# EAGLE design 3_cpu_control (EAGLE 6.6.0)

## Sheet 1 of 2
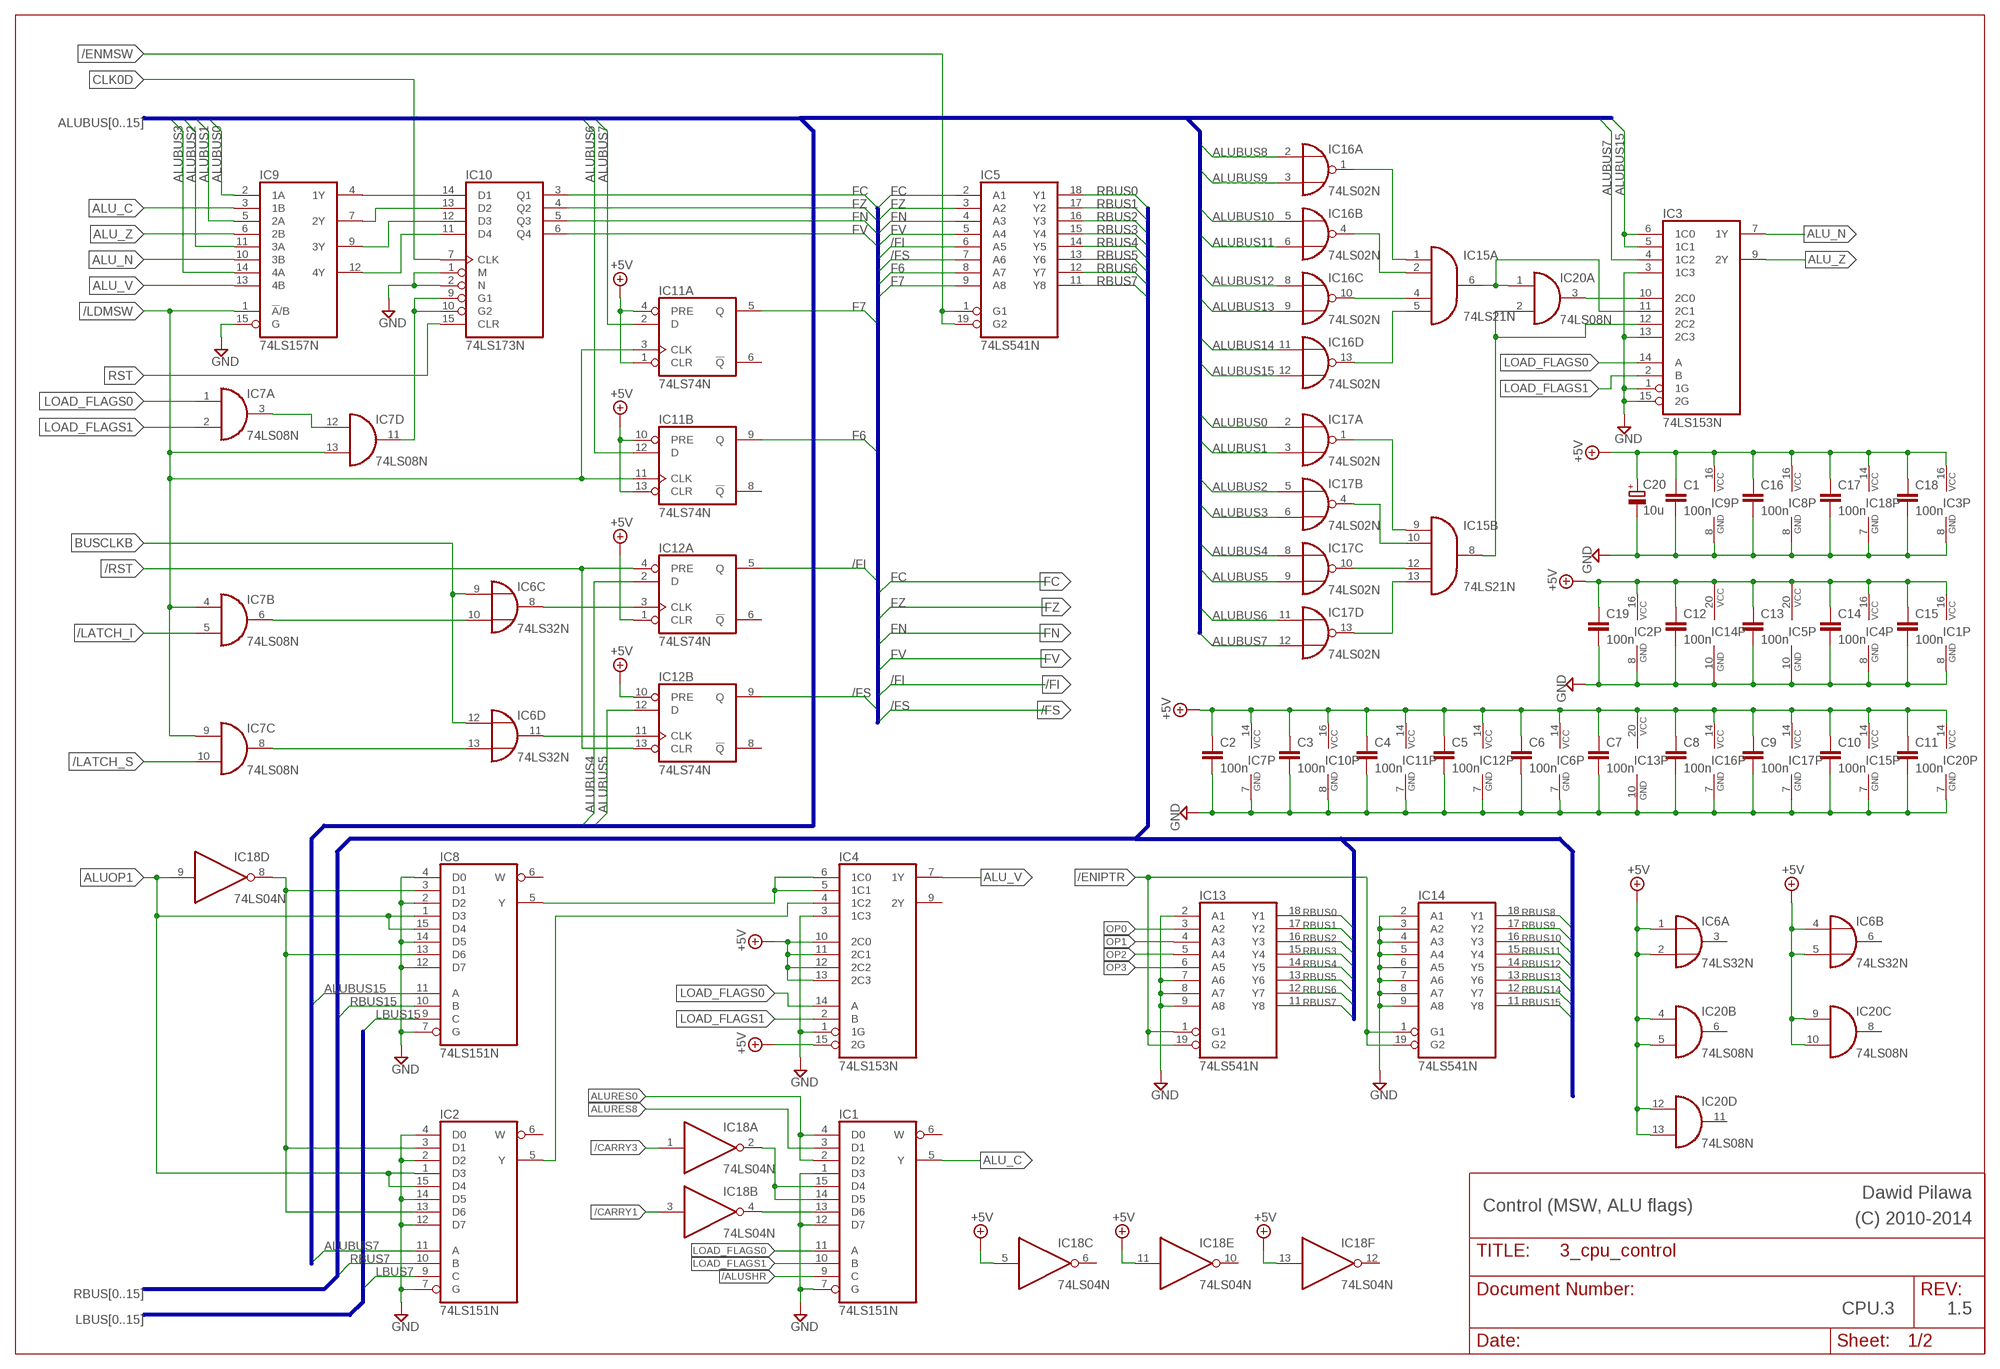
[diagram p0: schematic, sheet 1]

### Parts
C1  100n  C-EU050-024X044  [C050-024X044]
C2  100n  C-EU050-024X044  [C050-024X044]
C3  100n  C-EU050-024X044  [C050-024X044]
C4  100n  C-EU050-024X044  [C050-024X044]
C5  100n  C-EU050-024X044  [C050-024X044]
C6  100n  C-EU050-024X044  [C050-024X044]
C7  100n  C-EU050-024X044  [C050-024X044]
C8  100n  C-EU050-024X044  [C050-024X044]
C9  100n  C-EU050-024X044  [C050-024X044]
C10  100n  C-EU050-024X044  [C050-024X044]
C11  100n  C-EU050-024X044  [C050-024X044]
C12  100n  C-EU050-024X044  [C050-024X044]
C13  100n  C-EU050-024X044  [C050-024X044]
C14  100n  C-EU050-024X044  [C050-024X044]
C15  100n  C-EU050-024X044  [C050-024X044]
C16  100n  C-EU050-024X044  [C050-024X044]
C17  100n  C-EU050-024X044  [C050-024X044]
C18  100n  C-EU050-024X044  [C050-024X044]
C19  100n  C-EU050-024X044  [C050-024X044]
C20  10u  CPOL-EUE2.5-6  [E2,5-6]
IC1  74LS151N  [DIL16]
IC2  74LS151N  [DIL16]
IC3  74LS153N  [DIL16]
IC4  74LS153N  [DIL16]
IC5  74LS541N  [DIL20]
IC6  74LS32N  [DIL14]
IC7  74LS08N  [DIL14]
IC8  74LS151N  [DIL16]
IC9  74LS157N  [DIL16]
IC10  74LS173N  [DIL16]
IC11  74LS74N  [DIL14]
IC12  74LS74N  [DIL14]
IC13  74LS541N  [DIL20]
IC14  74LS541N  [DIL20]
IC15  74LS21N  [DIL14]
IC16  74LS02N  [DIL14]
IC17  74LS02N  [DIL14]
IC18  74LS04N  [DIL14]
IC20  74LS08N  [DIL14]

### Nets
+5V: C1.1 C2.1 C3.1 C4.1 C5.1 C6.1 C7.1 C8.1 C9.1 C10.1 C11.1 C12.1 C13.1 C14.1 C15.1 C16.1 C17.1 C18.1 C19.1 C20.+ IC1.16(VCC) IC2.16(VCC) IC3.16(VCC) IC4.10(2C0) IC4.11(2C1) IC4.12(2C2) IC4.13(2C3) IC4.15(2G) IC4.16(VCC) IC5.20(VCC) IC6.1(A:I0) IC6.2(A:I1) IC6.4(B:I0) IC6.5(B:I1) IC6.14(P:VCC) IC7.14(P:VCC) IC8.16(VCC) IC9.16(VCC) IC10.16(VCC) IC11.1(A:CLR) IC11.4(A:PRE) IC11.10(B:PRE) IC11.13(B:CLR) IC11.14(P:VCC) IC12.1(A:CLR) IC12.10(B:PRE) IC12.14(P:VCC) IC13.20(VCC) IC14.20(VCC) IC15.14(P:VCC) IC16.14(P:VCC) IC17.14(P:VCC) IC18.5(C:I) IC18.11(E:I) IC18.13(F:I) IC18.14(P:VCC) IC20.4(B:I0) IC20.5(B:I1) IC20.9(C:I0) IC20.10(C:I1) IC20.12(D:I0) IC20.13(D:I1) IC20.14(P:VCC) ; also sheet 2
/ALUSHR: IC1.9(C) ; also sheet 2
/CARRY1: IC18.3(B:I) ; also sheet 2
/CARRY3: IC18.1(A:I) ; also sheet 2
/ENIPTR: IC13.1(G1) IC13.19(G2) IC14.1(G1) IC14.19(G2) ; also sheet 2
/ENMSW: IC5.1(G1) IC5.19(G2) ; also sheet 2
/FI: IC5.6(A5) IC12.5(A:Q) ; also sheet 2
/FS: IC5.7(A6) IC12.9(B:Q) ; also sheet 2
/LATCH_I: IC7.5(B:I1) ; also sheet 2
/LATCH_S: IC7.10(C:I1) ; also sheet 2
/LDMSW: IC7.4(B:I0) IC7.9(C:I0) IC7.13(D:I1) IC9.1(!A!/B) IC11.3(A:CLK) IC11.11(B:CLK) ; also sheet 2
/RST: IC12.4(A:PRE) IC12.13(B:CLR) ; also sheet 2
ALU_C: IC1.5(Y) IC9.3(1B)
ALU_N: IC3.7(1Y) IC9.10(3B)
ALU_V: IC4.7(1Y) IC9.13(4B)
ALU_Z: IC3.9(2Y) IC9.6(2B)
ALUBUS0: IC9.2(1A) IC17.2(A:I0) ; also sheet 2
ALUBUS1: IC9.5(2A) IC17.3(A:I1) ; also sheet 2
ALUBUS2: IC9.11(3A) IC17.5(B:I0) ; also sheet 2
ALUBUS3: IC9.14(4A) IC17.6(B:I1) ; also sheet 2
ALUBUS4: IC12.2(A:D) IC17.8(C:I0) ; also sheet 2
ALUBUS5: IC12.12(B:D) IC17.9(C:I1) ; also sheet 2
ALUBUS6: IC11.12(B:D) IC17.11(D:I0) ; also sheet 2
ALUBUS7: IC2.11(A) IC3.4(1C2) IC11.2(A:D) IC17.12(D:I1) ; also sheet 2
ALUBUS8: IC16.2(A:I0) ; also sheet 2
ALUBUS9: IC16.3(A:I1) ; also sheet 2
ALUBUS10: IC16.5(B:I0) ; also sheet 2
ALUBUS11: IC16.6(B:I1) ; also sheet 2
ALUBUS12: IC16.8(C:I0) ; also sheet 2
ALUBUS13: IC16.9(C:I1) ; also sheet 2
ALUBUS14: IC16.11(D:I0) ; also sheet 2
ALUBUS15: IC3.5(1C1) IC3.6(1C0) IC8.11(A) IC16.12(D:I1) ; also sheet 2
ALUOP1: IC2.1(D3) IC2.15(D4) IC8.1(D3) IC8.15(D4) IC18.9(D:I) ; also sheet 2
ALURES0: IC1.2(D2) IC1.4(D0) ; also sheet 2
ALURES8: IC1.3(D1) ; also sheet 2
BUSCLKB: IC6.9(C:I0) IC6.12(D:I0) ; also sheet 2
CLK0D: IC10.7(CLK) ; also sheet 2
F6: IC5.8(A7) IC11.9(B:Q)
F7: IC5.9(A8) IC11.5(A:Q)
FC: IC5.2(A1) IC10.3(Q1) ; also sheet 2
FN: IC5.4(A3) IC10.5(Q3) ; also sheet 2
FV: IC5.5(A4) IC10.6(Q4) ; also sheet 2
FZ: IC5.3(A2) IC10.4(Q2) ; also sheet 2
GND: C1.2 C2.2 C3.2 C4.2 C5.2 C6.2 C7.2 C8.2 C9.2 C10.2 C11.2 C12.2 C13.2 C14.2 C15.2 C16.2 C17.2 C18.2 C19.2 C20.- IC1.1(D3) IC1.7(G) IC1.8(GND) IC1.12(D7) IC2.2(D2) IC2.4(D0) IC2.7(G) IC2.8(GND) IC2.12(D7) IC2.14(D5) IC3.1(1G) IC3.3(1C3) IC3.8(GND) IC3.13(2C3) IC3.15(2G) IC4.1(1G) IC4.3(1C3) IC4.8(GND) IC5.10(GND) IC6.7(P:GND) IC7.7(P:GND) IC8.2(D2) IC8.4(D0) IC8.7(G) IC8.8(GND) IC8.12(D7) IC8.14(D5) IC9.8(GND) IC9.15(G) IC10.1(M) IC10.2(N) IC10.8(GND) IC11.7(P:GND) IC12.7(P:GND) IC13.2(A1) IC13.7(A6) IC13.8(A7) IC13.9(A8) IC13.10(GND) IC14.2(A1) IC14.3(A2) IC14.4(A3) IC14.5(A4) IC14.6(A5) IC14.7(A6) IC14.8(A7) IC14.9(A8) IC14.10(GND) IC15.7(P:GND) IC16.7(P:GND) IC17.7(P:GND) IC18.7(P:GND) IC20.7(P:GND) ; also sheet 2
LBUS7: IC2.9(C) ; also sheet 2
LBUS15: IC8.9(C) ; also sheet 2
LOAD_FLAGS0: IC1.11(A) IC3.14(A) IC4.14(A) IC7.1(A:I0) ; also sheet 2
LOAD_FLAGS1: IC1.10(B) IC3.2(B) IC4.2(B) IC7.2(A:I1) ; also sheet 2
N$1: IC4.5(1C1) IC4.6(1C0) IC8.5(Y)
N$2: IC1.13(D6) IC18.4(B:O)
N$3: IC1.14(D5) IC1.15(D4) IC18.2(A:O)
N$6: IC15.1(A:I0) IC16.1(A:O)
N$7: IC15.2(A:I1) IC16.4(B:O)
N$8: IC15.4(A:I2) IC16.10(C:O)
N$9: IC15.5(A:I3) IC16.13(D:O)
N$10: IC15.9(B:I0) IC17.1(A:O)
N$11: IC15.10(B:I1) IC17.4(B:O)
N$12: IC15.12(B:I2) IC17.10(C:O)
N$13: IC15.13(B:I3) IC17.13(D:O)
N$14: IC3.11(2C1) IC15.6(A:O) IC20.1(A:I0)
N$15: IC3.12(2C2) IC15.8(B:O) IC20.2(A:I1)
N$16: IC3.10(2C0) IC20.3(A:O)
N$17: IC7.11(D:O) IC10.9(G1) IC10.10(G2)
N$19: IC2.5(Y) IC4.4(1C2)
N$21: IC2.3(D1) IC2.13(D6) IC8.3(D1) IC8.13(D6) IC18.8(D:O)
N$32: IC9.4(1Y) IC10.14(D1)
N$48: IC9.7(2Y) IC10.13(D2)
N$49: IC9.9(3Y) IC10.12(D3)
N$50: IC9.12(4Y) IC10.11(D4)
N$51: IC7.3(A:O) IC7.12(D:I0)
N$52: IC6.8(C:O) IC12.3(A:CLK)
N$53: IC6.11(D:O) IC12.11(B:CLK)
N$54: IC6.10(C:I1) IC7.6(B:O)
N$55: IC6.13(D:I1) IC7.8(C:O)
OP0: IC13.3(A2) ; also sheet 2
OP1: IC13.4(A3) ; also sheet 2
OP2: IC13.5(A4) ; also sheet 2
OP3: IC13.6(A5) ; also sheet 2
RBUS0: IC5.18(Y1) IC13.18(Y1) ; also sheet 2
RBUS1: IC5.17(Y2) IC13.17(Y2) ; also sheet 2
RBUS2: IC5.16(Y3) IC13.16(Y3) ; also sheet 2
RBUS3: IC5.15(Y4) IC13.15(Y4) ; also sheet 2
RBUS4: IC5.14(Y5) IC13.14(Y5) ; also sheet 2
RBUS5: IC5.13(Y6) IC13.13(Y6) ; also sheet 2
RBUS6: IC5.12(Y7) IC13.12(Y7) ; also sheet 2
RBUS7: IC2.10(B) IC5.11(Y8) IC13.11(Y8) ; also sheet 2
RBUS8: IC14.18(Y1) ; also sheet 2
RBUS9: IC14.17(Y2) ; also sheet 2
RBUS10: IC14.16(Y3) ; also sheet 2
RBUS11: IC14.15(Y4) ; also sheet 2
RBUS12: IC14.14(Y5) ; also sheet 2
RBUS13: IC14.13(Y6) ; also sheet 2
RBUS14: IC14.12(Y7) ; also sheet 2
RBUS15: IC8.10(B) IC14.11(Y8) ; also sheet 2
RST: IC10.15(CLR) ; also sheet 2
Unconnected: IC1.6(W) IC2.6(W) IC4.9(2Y) IC6.3(A:O) IC6.6(B:O) IC8.6(W) IC11.6(A:!Q) IC11.8(B:!Q) IC12.6(A:!Q) IC12.8(B:!Q) IC18.6(C:O) IC18.10(E:O) IC18.12(F:O) IC20.6(B:O) IC20.8(C:O) IC20.11(D:O)

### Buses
ALUBUS[0..15]
FC,FZ,FN,FV,/FI,/FS,F6,F7
RBUS[0..15]
LBUS[0..15]

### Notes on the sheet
- Dawid Pilawa
- Control (MSW, ALU flags) | (C) 2010-2014
- CPU.3 | 1.5

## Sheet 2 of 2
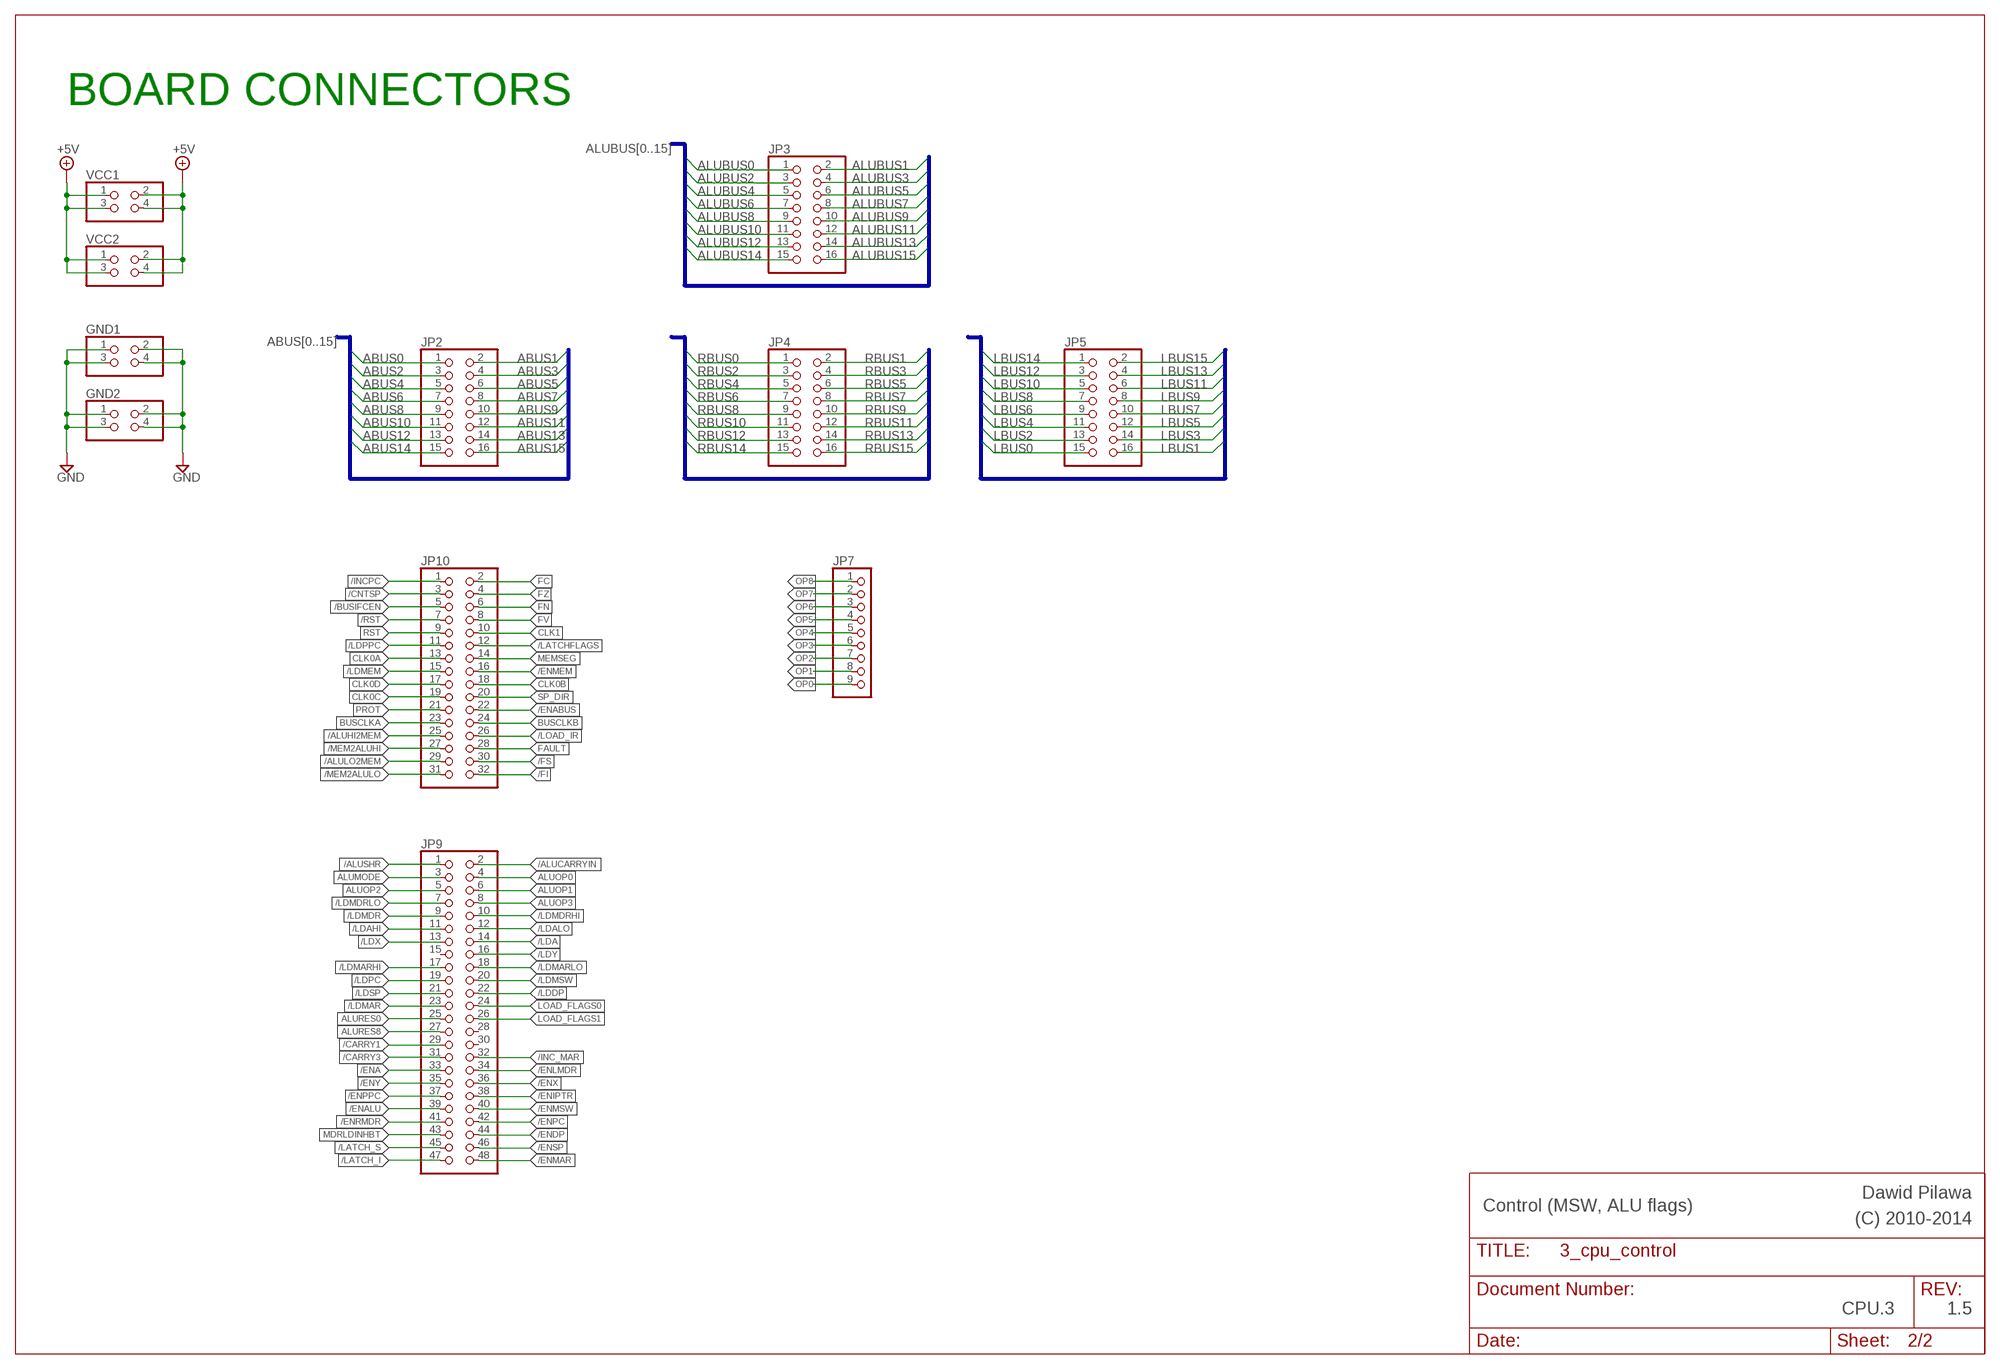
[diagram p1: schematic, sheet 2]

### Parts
GND1  PINHD-2X2  [2X02]
GND2  PINHD-2X2  [2X02]
JP2  PINHD-2X8  [2X08]
JP3  PINHD-2X8  [2X08]
JP4  PINHD-2X8  [2X08]
JP5  PINHD-2X8  [2X08]
JP7  PINHD-1X9  [1X09]
JP9  PINHD-2X24  [2X24]
JP10  PINHD-2X16  [2X16]
VCC1  PINHD-2X2  [2X02]
VCC2  PINHD-2X2  [2X02]

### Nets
+5V: VCC1.1 VCC1.2 VCC1.3 VCC1.4 VCC2.1 VCC2.2 VCC2.3 VCC2.4 ; also sheet 1
/ALUCARRYIN: JP9.2
/ALUHI2MEM: JP10.25
/ALULO2MEM: JP10.29
/ALUSHR: JP9.1 ; also sheet 1
/BUSIFCEN: JP10.5
/CARRY1: JP9.29 ; also sheet 1
/CARRY3: JP9.31 ; also sheet 1
/CNTSP: JP10.3
/ENA: JP9.33
/ENABUS: JP10.22
/ENALU: JP9.39
/ENDP: JP9.44
/ENIPTR: JP9.38 ; also sheet 1
/ENLMDR: JP9.34
/ENMAR: JP9.48
/ENMEM: JP10.16
/ENMSW: JP9.40 ; also sheet 1
/ENPC: JP9.42
/ENPPC: JP9.37
/ENRMDR: JP9.41
/ENSP: JP9.46
/ENX: JP9.36
/ENY: JP9.35
/FI: JP10.32 ; also sheet 1
/FS: JP10.30 ; also sheet 1
/INC_MAR: JP9.32
/INCPC: JP10.1
/LATCH_I: JP9.47 ; also sheet 1
/LATCH_S: JP9.45 ; also sheet 1
/LATCHFLAGS: JP10.12
/LDA: JP9.14
/LDAHI: JP9.11
/LDALO: JP9.12
/LDDP: JP9.22
/LDMAR: JP9.23
/LDMARHI: JP9.17
/LDMARLO: JP9.18
/LDMDR: JP9.9
/LDMDRHI: JP9.10
/LDMDRLO: JP9.7
/LDMEM: JP10.15
/LDMSW: JP9.20 ; also sheet 1
/LDPC: JP9.19
/LDPPC: JP10.11
/LDSP: JP9.21
/LDX: JP9.13
/LDY: JP9.16
/LOAD_IR: JP10.26
/MEM2ALUHI: JP10.27
/MEM2ALULO: JP10.31
/RST: JP10.7 ; also sheet 1
ABUS0: JP2.1
ABUS1: JP2.2
ABUS2: JP2.3
ABUS3: JP2.4
ABUS4: JP2.5
ABUS5: JP2.6
ABUS6: JP2.7
ABUS7: JP2.8
ABUS8: JP2.9
ABUS9: JP2.10
ABUS10: JP2.11
ABUS11: JP2.12
ABUS12: JP2.13
ABUS13: JP2.14
ABUS14: JP2.15
ABUS15: JP2.16
ALUBUS0: JP3.1 ; also sheet 1
ALUBUS1: JP3.2 ; also sheet 1
ALUBUS2: JP3.3 ; also sheet 1
ALUBUS3: JP3.4 ; also sheet 1
ALUBUS4: JP3.5 ; also sheet 1
ALUBUS5: JP3.6 ; also sheet 1
ALUBUS6: JP3.7 ; also sheet 1
ALUBUS7: JP3.8 ; also sheet 1
ALUBUS8: JP3.9 ; also sheet 1
ALUBUS9: JP3.10 ; also sheet 1
ALUBUS10: JP3.11 ; also sheet 1
ALUBUS11: JP3.12 ; also sheet 1
ALUBUS12: JP3.13 ; also sheet 1
ALUBUS13: JP3.14 ; also sheet 1
ALUBUS14: JP3.15 ; also sheet 1
ALUBUS15: JP3.16 ; also sheet 1
ALUMODE: JP9.3
ALUOP0: JP9.4
ALUOP1: JP9.6 ; also sheet 1
ALUOP2: JP9.5
ALUOP3: JP9.8
ALURES0: JP9.25 ; also sheet 1
ALURES8: JP9.27 ; also sheet 1
BUSCLKA: JP10.23
BUSCLKB: JP10.24 ; also sheet 1
CLK0A: JP10.13
CLK0B: JP10.18
CLK0C: JP10.19
CLK0D: JP10.17 ; also sheet 1
CLK1: JP10.10
FAULT: JP10.28
FC: JP10.2 ; also sheet 1
FN: JP10.6 ; also sheet 1
FV: JP10.8 ; also sheet 1
FZ: JP10.4 ; also sheet 1
GND: GND1.1 GND1.2 GND1.3 GND1.4 GND2.1 GND2.2 GND2.3 GND2.4 ; also sheet 1
LBUS0: JP5.15
LBUS1: JP5.16
LBUS2: JP5.13
LBUS3: JP5.14
LBUS4: JP5.11
LBUS5: JP5.12
LBUS6: JP5.9
LBUS7: JP5.10 ; also sheet 1
LBUS8: JP5.7
LBUS9: JP5.8
LBUS10: JP5.5
LBUS11: JP5.6
LBUS12: JP5.3
LBUS13: JP5.4
LBUS14: JP5.1
LBUS15: JP5.2 ; also sheet 1
LOAD_FLAGS0: JP9.24 ; also sheet 1
LOAD_FLAGS1: JP9.26 ; also sheet 1
MDRLDINHBT: JP9.43
MEMSEG: JP10.14
OP0: JP7.9 ; also sheet 1
OP1: JP7.8 ; also sheet 1
OP2: JP7.7 ; also sheet 1
OP3: JP7.6 ; also sheet 1
OP4: JP7.5
OP5: JP7.4
OP6: JP7.3
OP7: JP7.2
OP8: JP7.1
PROT: JP10.21
RBUS0: JP4.1 ; also sheet 1
RBUS1: JP4.2 ; also sheet 1
RBUS2: JP4.3 ; also sheet 1
RBUS3: JP4.4 ; also sheet 1
RBUS4: JP4.5 ; also sheet 1
RBUS5: JP4.6 ; also sheet 1
RBUS6: JP4.7 ; also sheet 1
RBUS7: JP4.8 ; also sheet 1
RBUS8: JP4.9 ; also sheet 1
RBUS9: JP4.10 ; also sheet 1
RBUS10: JP4.11 ; also sheet 1
RBUS11: JP4.12 ; also sheet 1
RBUS12: JP4.13 ; also sheet 1
RBUS13: JP4.14 ; also sheet 1
RBUS14: JP4.15 ; also sheet 1
RBUS15: JP4.16 ; also sheet 1
RST: JP10.9 ; also sheet 1
SP_DIR: JP10.20
Unconnected: JP9.15 JP9.28 JP9.30

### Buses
ALUBUS[0..15]
RBUS[0..15]
LBUS[0..15]
ABUS[0..15]

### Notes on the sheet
- BOARD CONNECTORS
- Dawid Pilawa
- Control (MSW, ALU flags) | (C) 2010-2014
- CPU.3 | 1.5

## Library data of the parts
C1-C19 = rcl:C-EU: CAPACITOR, European symbol
C20 = rcl:CPOL-EU: POLARIZED CAPACITOR, European symbol
GND1 GND2 VCC1 VCC2 = pinhead:PINHD-2X2: PIN HEADER
IC1 IC2 IC8 = 74xx-eu:74*151: Data SELECTOR/MULTIPLEXER
IC3 IC4 = 74xx-eu:74*153: Dual 4-line to 1-line data SELECTOR/MULTIPLEXER
IC5 IC13 IC14 = 74xx-us:74*541: Octal BUFFER and LINE DRIVER, 3-state
IC6 = 74xx-eu:74*32: Quad 2-input OR gate
IC7 IC20 = 74xx-eu:74*08: Quad 2-input AND gate
IC9 = 74xx-eu:74*157: Quadruple 2-line to 1-line data SELECTOR/MULTIPLEXER
IC10 = 74xx-eu:74*173: 4-bit D type REGISTER, 3-state
IC11 IC12 = 74xx-eu:74*74: Dual D type positive edge triggered FLIP FLOP, preset and clear
IC15 = 74xx-eu:74*21: Dual 4-input AND gate
IC16 IC17 = 74xx-eu:74*02: Quad 2-input NOR gate
IC18 = 74xx-eu:74*04: Hex INVERTER
JP2-JP5 = pinhead:PINHD-2X8: PIN HEADER
JP7 = pinhead:PINHD-1X9: PIN HEADER
JP9 = pinhead:PINHD-2X24: PIN HEADER
JP10 = pinhead:PINHD-2X16: PIN HEADER

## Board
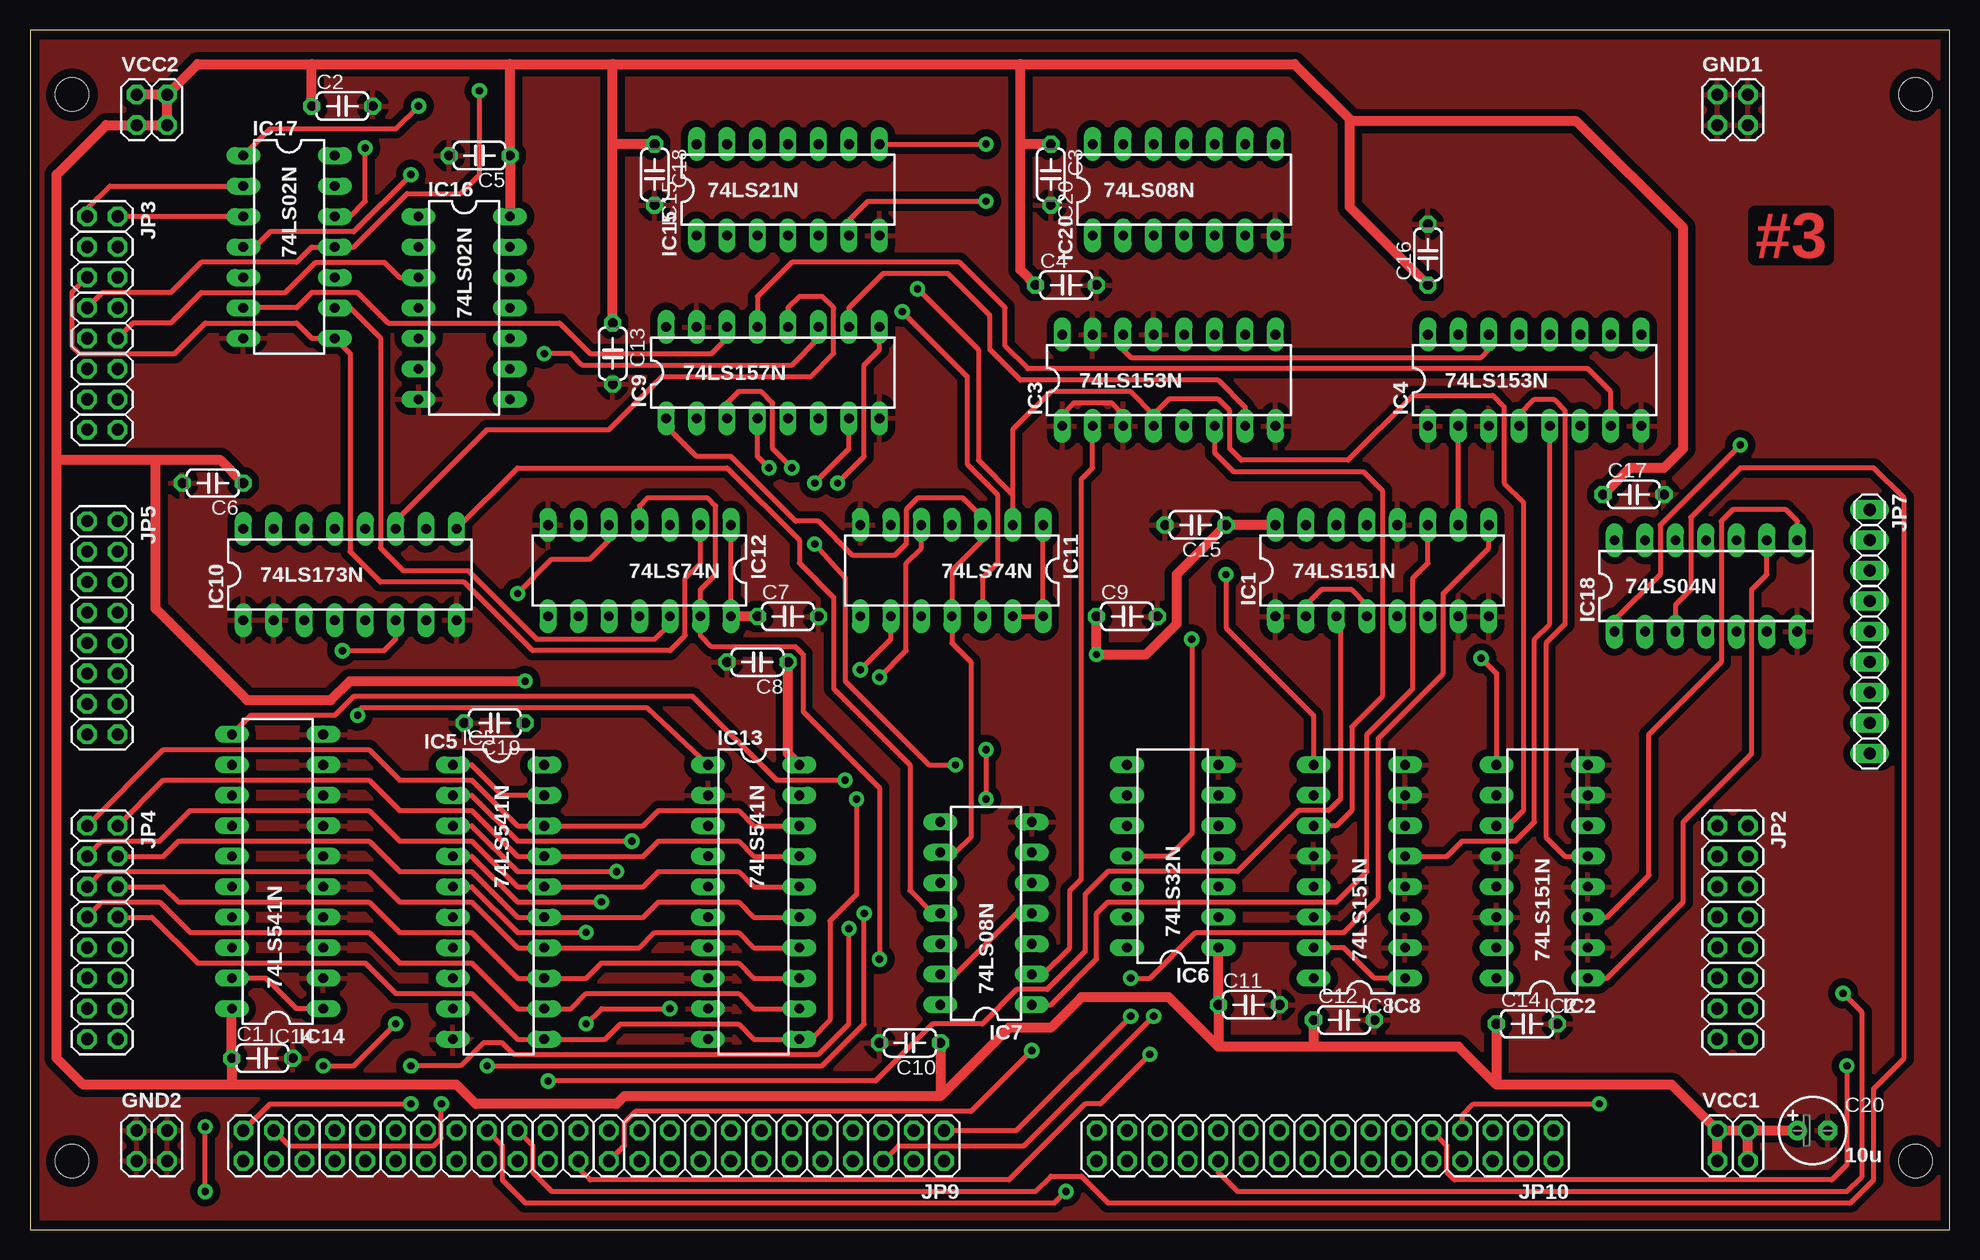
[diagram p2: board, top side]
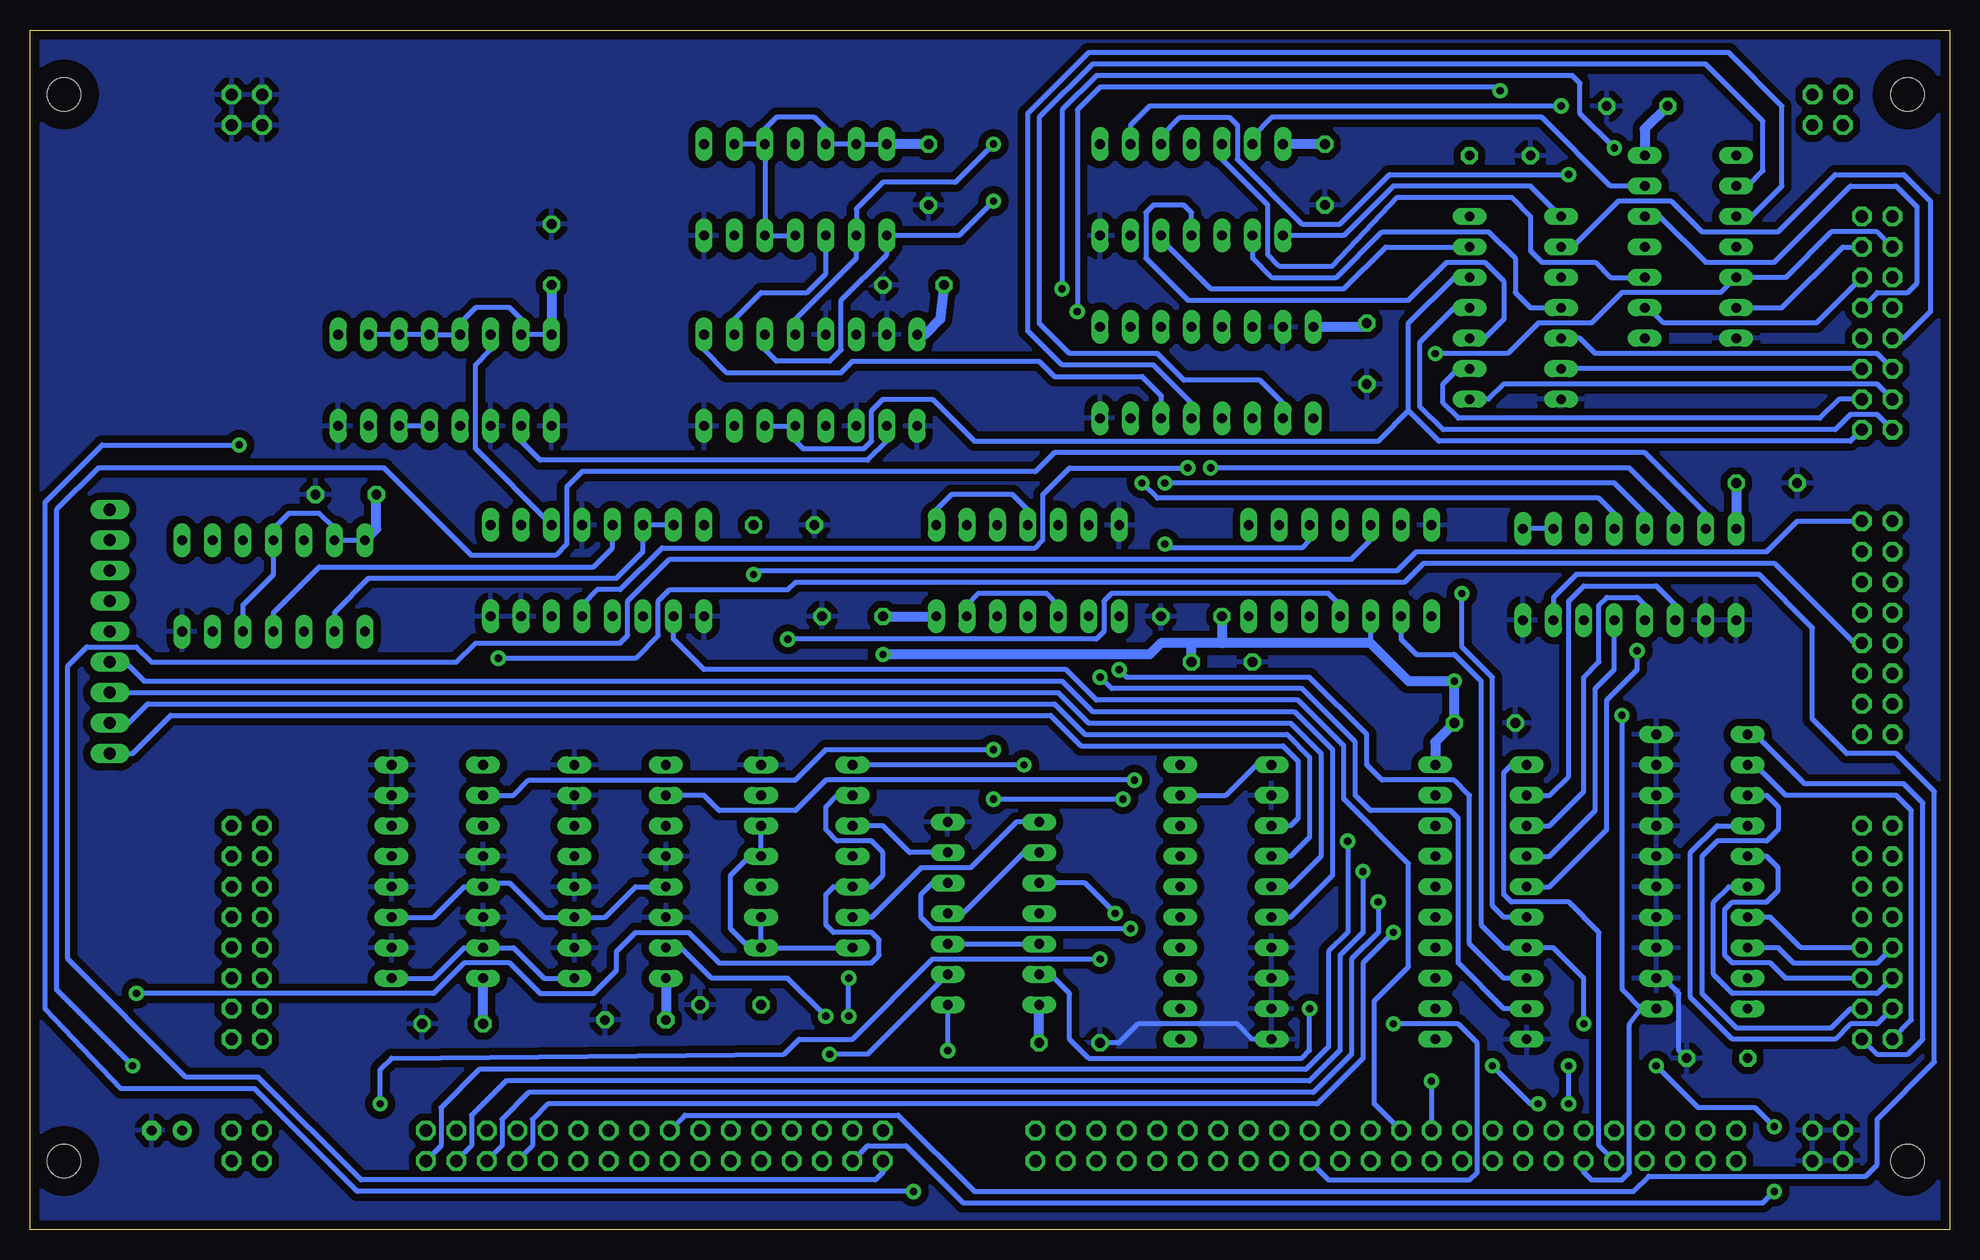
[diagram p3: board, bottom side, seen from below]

Size 160 x 100 mm. Coordinates in mm from the lower left corner, seen from the top.
Outline: 0,0 160,0 160,100 0,100 0,0
Copper layers (1*16): Top 0.035mm / dielectric 1.5mm / Bottom 0.035mm
Design rules "homebrew_pcb": minimum track width 16mil, minimum drill 24mil, track to track 16mil, track to pad 10mil, pad to pad 10mil, via to via 10mil, smd to smd 8mil, copper to edge 30mil, drill to drill 10mil, minimum pad ring 12mil, minimum via ring 12mil, stop-mask expansion 4mil, vias tented up to drill 0mil, thermal gap 24mil
Holes 2.79 mm at 3.49,94.61 3.49,5.71 157.16,5.71 157.16,94.61
bRestrict: area 1.2,92.3 to 5.8,96.9; area 1.2,3.4 to 5.8,8; area 154.9,3.4 to 159.4,8; area 154.9,92.3 to 159.4,96.9
vRestrict: area 1.2,92.3 to 5.8,96.9; area 154.9,3.4 to 159.4,8; area 154.9,92.3 to 159.4,96.9; area 1.2,3.4 to 5.8,8

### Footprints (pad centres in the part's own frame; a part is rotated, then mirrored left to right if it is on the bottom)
C050-024X044 = drill 0.813 octagon: 1 -2.54,0; 2 2.54,0
E2,5-6 = drill 0.813 pad 1.6: + -1.27,0 | drill 0.813 pad 1.6 octagon: - 1.27,0
2X02 = drill 1.016 octagon: 1 -1.27,-1.27; 2 -1.27,1.27; 3 1.27,-1.27; 4 1.27,1.27
DIL16 = drill 0.813 long: 1 -8.89,-3.81; 2 -6.35,-3.81; 3 -3.81,-3.81; 4 -1.27,-3.81; 5 1.27,-3.81; 6 3.81,-3.81; 7 6.35,-3.81; 8 8.89,-3.81; 9 8.89,3.81; 10 6.35,3.81; 11 3.81,3.81; 12 1.27,3.81; 13 -1.27,3.81; 14 -3.81,3.81; 15 -6.35,3.81; 16 -8.89,3.81
DIL20 = drill 0.813 long: 1 -11.43,-3.81; 2 -8.89,-3.81; 3 -6.35,-3.81; 4 -3.81,-3.81; 5 -1.27,-3.81; 6 1.27,-3.81; 7 3.81,-3.81; 8 6.35,-3.81; 9 8.89,-3.81; 10 11.43,-3.81; 11 11.43,3.81; 12 8.89,3.81; 13 6.35,3.81; 14 3.81,3.81; 15 1.27,3.81; 16 -1.27,3.81; 17 -3.81,3.81; 18 -6.35,3.81; 19 -8.89,3.81; 20 -11.43,3.81
DIL14 = drill 0.813 long: 1 -7.62,-3.81; 2 -5.08,-3.81; 3 -2.54,-3.81; 4 0,-3.81; 5 2.54,-3.81; 6 5.08,-3.81; 7 7.62,-3.81; 8 7.62,3.81; 9 5.08,3.81; 10 2.54,3.81; 11 0,3.81; 12 -2.54,3.81; 13 -5.08,3.81; 14 -7.62,3.81
2X08 = drill 1.016 octagon: 1 -8.89,-1.27; 2 -8.89,1.27; 3 -6.35,-1.27; 4 -6.35,1.27; 5 -3.81,-1.27; 6 -3.81,1.27; 7 -1.27,-1.27; 8 -1.27,1.27; 9 1.27,-1.27; 10 1.27,1.27; 11 3.81,-1.27; 12 3.81,1.27; 13 6.35,-1.27; 14 6.35,1.27; 15 8.89,-1.27; 16 8.89,1.27
1X09 = drill 1.016 long: 1 -10.16,0; 2 -7.62,0; 3 -5.08,0; 4 -2.54,0; 5 0,0; 6 2.54,0; 7 5.08,0; 8 7.62,0; 9 10.16,0
2X24 = drill 1.016 octagon: 1 -27.94,-1.27; 2 -27.94,1.27; 3 -25.4,-1.27; 4 -25.4,1.27; 5 -22.86,-1.27; 6 -22.86,1.27; 7 -20.32,-1.27; 8 -20.32,1.27; 9 -17.78,-1.27; 10 -17.78,1.27; 11 -15.24,-1.27; 12 -15.24,1.27; 13 -12.7,-1.27; 14 -12.7,1.27; 15 -10.16,-1.27; 16 -10.16,1.27; 17 -7.62,-1.27; 18 -7.62,1.27; 19 -5.08,-1.27; 20 -5.08,1.27; 21 -2.54,-1.27; 22 -2.54,1.27; 23 0,-1.27; 24 0,1.27; 25 2.54,-1.27; 26 2.54,1.27; 27 5.08,-1.27; 28 5.08,1.27; 29 7.62,-1.27; 30 7.62,1.27; 31 10.16,-1.27; 32 10.16,1.27; 33 12.7,-1.27; 34 12.7,1.27; 35 15.24,-1.27; 36 15.24,1.27; 37 17.78,-1.27; 38 17.78,1.27; 39 20.32,-1.27; 40 20.32,1.27; 41 22.86,-1.27; 42 22.86,1.27; 43 25.4,-1.27; 44 25.4,1.27; 45 27.94,-1.27; 46 27.94,1.27; 47 30.48,-1.27; 48 30.48,1.27
2X16 = drill 1.016 octagon: 1 -19.05,-1.27; 2 -19.05,1.27; 3 -16.51,-1.27; 4 -16.51,1.27; 5 -13.97,-1.27; 6 -13.97,1.27; 7 -11.43,-1.27; 8 -11.43,1.27; 9 -8.89,-1.27; 10 -8.89,1.27; 11 -6.35,-1.27; 12 -6.35,1.27; 13 -3.81,-1.27; 14 -3.81,1.27; 15 -1.27,-1.27; 16 -1.27,1.27; 17 1.27,-1.27; 18 1.27,1.27; 19 3.81,-1.27; 20 3.81,1.27; 21 6.35,-1.27; 22 6.35,1.27; 23 8.89,-1.27; 24 8.89,1.27; 25 11.43,-1.27; 26 11.43,1.27; 27 13.97,-1.27; 28 13.97,1.27; 29 16.51,-1.27; 30 16.51,1.27; 31 19.05,-1.27; 32 19.05,1.27

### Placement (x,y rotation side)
C1  19.37,14.29 0 top
C2  26.04,93.66 0 top
C3  85.09,87.95 270 top
C4  86.36,78.74 0 top
C5  37.47,89.53 180 top
C6  15.24,62.23 180 top
C7  63.18,51.12 0 top
C8  60.64,47.31 180 top
C9  91.44,51.12 0 top
C10  73.34,15.56 180 top
C11  101.6,18.73 0 top
C12  109.54,17.46 0 top
C13  48.58,73.03 270 top
C14  124.78,17.14 0 top
C15  97.16,58.74 180 top
C16  116.52,81.28 90 top
C17  133.67,61.28 0 top
C18  52.07,87.95 270 top
C19  38.73,42.23 180 top
C20  148.59,8.26 0 top
GND1  141.92,93.34 0 top
GND2  10.16,6.99 0 top
IC1  112.71,54.93 0 top
IC2  126.05,29.84 90 top
IC3  94.93,70.8 0 top
IC4  125.41,70.8 0 top
IC5  39.05,27.3 270 top
IC6  95.25,31.11 90 top
IC7  79.69,26.35 90 top
IC8  110.81,29.84 90 top
IC9  61.91,71.44 0 top
IC10  26.67,54.61 0 top
IC11  76.83,54.93 180 top
IC12  50.8,54.93 180 top
IC13  60.33,27.3 270 top
IC14  20.64,29.84 90 top
IC15  63.18,86.68 0 top
IC16  36.2,76.83 270 top
IC17  21.59,81.92 270 top
IC18  139.7,53.66 0 top
IC20  96.2,86.68 0 top
JP2  141.92,24.77 270 top
JP3  6.03,75.56 270 top
JP4  6.03,24.77 270 top
JP5  6.03,50.16 270 top
JP7  153.35,49.85 270 top
JP9  48.26,6.99 180 top
JP10  107.95,6.99 180 top
VCC1  141.92,6.99 0 top
VCC2  10.16,93.34 0 top

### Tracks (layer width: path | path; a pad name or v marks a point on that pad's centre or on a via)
+5V  (via drill 0.61 pad 1.27)
  Top 0.406: IC12.14 IC12.1 | IC11.1 IC11.14 IC11.13
  Top 0.813: VCC1.2 136.84,12.06 122.24,12.06 | 75.88,11.11 49.53,11.11 48.9,10.48 37.15,10.48 35.56,12.06 16.83,12.06 | 16.83,12.06 4.45,12.06 2.22,14.29 2.22,64.14 | 2.22,64.14 2.22,87.95 6.35,92.08 VCC2.1 VCC2.3 VCC2.4 | VCC2.4 13.97,97.16 23.5,97.16 | 23.5,97.16 40.01,97.16 | 40.01,97.16 48.58,97.16 | 48.58,97.16 82.55,97.16 | 82.55,97.16 105.41,97.16 110.01,92.55 | C13.1 48.58,90.49 | 48.58,90.49 48.58,97.16 | C18.1 48.58,90.49 | C2.1 23.5,97.16 | 40.01,97.16 C5.1 IC16.14 | 110.01,92.55 110.17,92.39 128.91,92.39 137.79,83.5 137.79,65.09 136.21,63.5 133.35,63.5 C17.1 | 82.55,90.49 82.55,97.16 | C3.1 82.55,90.49 | C7.1 IC12.14 | IC1.16 C15.1 95.57,54.61 95.57,50.48 93.03,47.94 v88.9,47.94 C9.1 | VCC2.4 VCC2.2 | VCC1.1 VCC1.2 | VCC1.3 VCC1.4 | VCC1.2 VCC1.4 | VCC1.4 C20.+ | C10.1 75.88,11.11 | IC6.1 C11.1 99.06,15.24 | C14.1 122.24,12.06 | 82.55,90.49 82.55,80.01 C4.1 | C16.1 110.01,85.25 110.01,92.55 | C6.1 15.88,64.14 10.48,64.14 | 10.48,64.14 2.22,64.14 | 10.48,64.14 10.48,51.75 18.1,44.13 25.08,44.13 26.67,45.72 v41.27,45.72 | IC13.20 63.18,39.69 C8.1 | 122.24,12.06 119.06,15.24 107,15.24 | 107,15.24 99.06,15.24 | 99.06,15.24 94.93,19.37 87.63,19.37 85.09,16.83 81.6,16.83 75.88,11.11 | C12.1 107,15.24 | IC14.20 C1.1 16.83,12.06
  Bottom 0.406: IC18.14 IC18.13 134.62,58.42 135.89,59.69 138.43,59.69 139.7,58.42 IC18.11 139.7,54.61 142.24,52.07 IC18.5 | IC20.14 IC20.13 IC20.12 93.66,91.76 94.61,92.71 97.79,92.71 98.74,91.76 IC20.10 | IC20.10 IC20.9 | IC20.10 IC20.5 IC20.4 | IC4.16 IC4.15 119.06,75.88 120.02,76.83 122.87,76.83 124.14,75.56 IC4.13 IC4.12 IC4.11 IC4.10 | IC11.10 74.3,52.07 75.25,53.02 80.96,53.02 81.92,52.07 IC11.13 | IC11.4 76.83,60.01 78.11,61.28 83.19,61.28 84.45,60.01 IC11.1 | IC12.10 48.26,48.9 | IC6.1 IC6.14 | IC6.5 IC6.4 100.01,31.11 101.6,29.53 101.6,25.08 100.01,23.5 IC6.1 | IC6.1 IC6.2
  Bottom 0.813: C13.1 48.9,75.25 IC9.16 | C18.1 IC15.14 | C2.1 25.4,91.76 IC17.14 | C16.1 IC4.16 | C3.1 IC20.14 | C9.1 IC11.14 | C10.1 IC7.14 | C14.1 IC2.16 | IC18.14 131.13,58.42 C17.1 | C4.1 84.14,75.88 85.41,74.61 IC3.16 | C6.1 IC10.16 | IC5.20 42.86,40.64 C19.1 v41.27,45.72 45.09,45.72 48.26,48.9 60.64,48.9 | 60.64,48.9 63.18,48.9 | 63.18,48.9 65.72,48.9 66.67,47.94 v88.9,47.94 | C7.1 60.64,48.9 | C8.1 63.18,48.9 | IC8.16 C12.1
/ALUSHR  (via drill 0.61 pad 1.27)
  Top 0.406: JP9.1 82.23,8.26 v91.76,17.78 | v91.76,20.95 93.34,20.95 97.16,24.77 109.54,24.77 112.39,27.62 112.39,40.96 117.79,46.35 117.79,53.02 121.6,56.83 IC1.9
  Bottom 0.406: v91.76,17.78 v91.76,20.95
/CARRY1
  Top 0.406: JP9.29 41.91,6.99 41.91,4.76 43.5,3.17 83.82,3.17 85.09,4.45 87.63,4.45 89.85,2.22 151.76,2.22 153.67,4.13 153.67,11.75 156.21,14.29 156.21,60.96 153.67,63.5 142.56,63.5 138.43,59.37 138.43,53.34 137.16,52.07 IC18.3
/CARRY3  (via drill 0.61 pad 1.27)
  Top 0.406: JP9.31 39.37,6.99 39.37,4.13 41.27,2.22 85.41,2.22 v86.36,3.17 | v142.56,65.41 135.89,58.74 135.89,54.61 132.08,50.8 IC18.1
  Bottom 0.406: v86.36,3.17 132.72,3.17 141.29,11.75 152.4,11.75 158.75,18.41 158.75,60.64 153.99,65.41 v142.56,65.41
/ENIPTR  (via drill 0.61 pad 1.27)
  Top 0.406: IC13.1 51.44,43.5 27.62,43.5 v27.3,42.86 | IC14.1 22.23,18.41 19.68,20.95 IC14.19
  Bottom 0.406: 30.48,6.35 JP9.38 30.48,4.76 29.84,4.13 27.3,4.13 26.67,4.76 26.67,17.14 25.72,18.41 | IC13.19 60.33,36.2 57.78,38.73 IC13.1 | v27.3,42.86 27.3,20 25.72,18.41 | 25.72,18.41 IC14.1
/ENMSW
  Top 0.406: IC5.19 39.37,36.2 36.83,38.73 IC5.1
  Bottom 0.406: JP9.40 29.21,6.99 29.21,24.77 31.75,27.3 36.51,27.3 37.15,27.94 37.15,38.1 36.51,38.73 IC5.1
/FI  (via drill 0.61 pad 1.27)
  Top 0.406: v40.64,53.02 43.5,55.88 46.67,55.88 48.26,57.47 IC12.5
  Bottom 0.406: JP10.32 88.9,4.76 89.53,4.13 132.4,4.13 140.97,12.7 147,12.7 156.84,22.54 156.84,46.99 155.26,48.58 151.13,48.58 149.86,47.31 124.46,47.31 122.87,48.9 110.81,48.9 110.17,49.53 110.17,52.39 106.68,55.88 49.85,55.88 48.26,57.47 IC12.5 | IC5.6 37.15,26.04 38.1,26.99 38.1,46.04 40.64,48.58 v40.64,53.02
/FS  (via drill 0.61 pad 1.27)
  Top 0.406: v14.61,3.17 v14.61,8.57 | v24.45,13.65 26.99,13.65 v30.48,17.14
  Bottom 0.406: IC12.9 45.72,49.21 44.45,47.94 41.27,47.94 39.05,45.72 39.05,25.4 37.15,23.5 IC5.7 33.02,23.5 30.48,20.95 v30.48,17.14 | v14.61,3.17 15.56,2.22 81.6,2.22 82.23,2.22 87,6.99 90.17,6.99 JP10.30 | v14.61,8.57 16.19,10.16 20.95,10.16 v24.45,13.65
/LATCH_I  (via drill 0.61 pad 1.27)
  Top 0.406: JP9.47 20,10.48 v31.75,10.48 | v68.26,25.08 68.26,17.14 65.72,14.61 40.32,14.61 39.37,15.56 37.78,15.56 35.88,13.65 v31.75,13.65
  Bottom 0.406: v31.75,10.48 v31.75,13.65 | v68.26,25.08 84.77,25.08 85.72,26.04 85.72,27.94 84.77,28.89 IC7.5
/LATCH_S  (via drill 0.61 pad 1.27)
  Top 0.406: JP9.45 21.59,6.99 33.66,6.99 34.29,7.62 v34.29,10.48 | v38.1,13.65 66.04,13.65 69.53,17.14 v69.53,26.35
  Bottom 0.406: v34.29,10.48 34.92,10.48 v38.1,13.65 | v69.53,26.35 72.07,28.89 IC7.10
/LDMSW  (via drill 0.61 pad 1.27)
  Top 0.406: IC9.1 53.02,66.99 55.56,64.45 58.42,64.45 63.82,59.05 65.72,59.05 68.58,56.2 72.07,56.2 73.03,57.15 73.03,60.01 73.98,60.96 77.79,60.96 79.38,59.37 IC11.3 79.38,57.47 76.83,54.93 IC11.11 76.83,48.9 78.42,47.31 78.42,32.7 77.15,31.43 IC7.9 | IC7.13 77.15,21.27 82.23,26.35 IC7.4 | v46.35,17.14 47.62,18.41 v53.34,18.41
  Bottom 0.406: IC7.4 82.23,26.35 77.15,31.43 IC7.9 | JP9.20 51.75,4.13 40.01,4.13 39.37,4.76 39.37,15.56 40.96,17.14 v46.35,17.14 | v53.34,18.41 53.34,14.92 53.98,14.29 71.75,14.29 73.34,15.88 73.34,19.68 74.93,21.27 IC7.13
/RST  (via drill 0.61 pad 1.27)
  Top 0.406: IC12.4 50.8,60.33 51.44,60.96 56.52,60.96 57.15,60.33 57.15,54.61 55.88,53.34 IC12.13 55.88,49.53 56.83,48.58 63.82,48.58 64.45,47.94 64.45,43.18 70.8,36.83 v70.8,22.54 | JP10.7 119.38,9.53 120.33,10.48 v130.81,10.48
  Bottom 0.406: v130.81,10.48 130.81,13.34 129.86,14.29 97.16,14.61 95.89,15.88 91.44,15.88 84.77,22.54 v70.8,22.54
ALU_C  (via drill 0.61 pad 1.27)
  Top 0.406: v63.5,63.5 61.91,65.09 61.91,68.9 60.96,69.85 59.05,69.85 58.1,68.9 IC9.3
  Bottom 0.406: v63.5,63.5 73.34,63.5 75.56,61.28 75.56,57.47 76.2,56.83 107.31,56.83 110.81,53.34 112.71,53.34 113.98,52.07 IC1.5
ALU_N
  Top 0.406: IC9.10 68.26,76.83 71.12,79.69 76.52,79.69 80.01,76.2 80.01,73.34 82.55,70.8 99.06,70.8 101.28,68.58 IC3.7
ALU_V
  Top 0.406: IC4.7 131.76,69.85 129.86,71.75 83.19,71.75 81.28,73.66 81.28,76.83 77.47,80.64 63.5,80.64 60.64,77.79 IC9.13
ALU_Z
  Bottom 0.406: IC9.6 65.72,69.53 67.31,71.12 74.61,71.12 75.88,72.39 91.44,72.39 92.39,71.44 101.92,71.44 103.82,73.34 IC3.9
ALUBUS0
  Top 0.406: JP3.1 4.76,85.09 6.67,87 IC17.2
  Bottom 0.406: IC9.2 55.56,68.9 57.47,70.8 63.82,70.8 66.04,73.03 73.34,73.03 75.88,75.56 75.88,92.71 71.44,97.16 20.32,97.16 15.56,92.39 15.56,88.27 16.83,87 IC17.2
ALUBUS1
  Top 0.406: IC17.3 JP3.2
  Bottom 0.406: IC9.5 63.18,68.9 66.36,72.07 73.98,72.07 76.83,74.93 76.83,93.03 71.75,98.11 18.41,98.11 13.97,93.66 13.97,87 16.51,84.45 IC17.3
ALUBUS2  (via drill 0.61 pad 1.27)
  Top 0.406: IC9.11 65.72,74.3 63.5,72.07 46.04,72.07 45.09,73.03 v42.86,73.03
  Bottom 0.406: JP3.3 6.03,83.19 9.84,83.19 13.65,79.38 IC17.5 19.05,78.11 27.3,78.11 29.84,75.56 34.29,75.56 36.83,73.03 v42.86,73.03
ALUBUS3
  Top 0.406: IC9.14 58.1,74.3 56.83,73.03 46.67,73.03 44.13,75.56 29.84,75.56 27.3,78.11 23.5,78.11 22.23,76.83 IC17.6
  Bottom 0.406: IC17.6 13.97,76.83 8.89,81.92 JP3.4
ALUBUS4
  Top 0.406: JP3.5 3.49,78.11 3.49,73.66 4.13,73.03 12.06,73.03 14.61,75.56 22.23,75.56 23.5,74.3 IC17.8 26.67,73.03 26.67,56.52 29.21,53.98 36.2,53.98 41.91,48.26 53.34,48.26 54.61,49.53 54.61,54.29 55.88,55.56 IC12.2
ALUBUS5
  Top 0.406: IC17.9 26.67,76.83 29.21,74.3 29.21,56.83 31.11,54.93 36.51,54.93 42.23,49.21 52.07,49.21 53.34,50.48 IC12.12
  Bottom 0.406: JP3.6 11.11,75.56 23.81,75.56 25.08,76.83 IC17.9
ALUBUS6  (via drill 0.61 pad 1.27)
  Top 0.406: JP3.7 6.03,78.11 11.75,78.11 14.29,80.64 22.23,80.64 23.5,81.92 IC17.11 26.99,81.92 31.43,86.36 35.88,86.36 37.47,87.95 v37.47,94.93 | v72.71,76.52 78.11,71.12 78.11,63.82 80.64,61.28 80.64,55.56 79.38,54.29 IC11.12
  Bottom 0.406: v37.47,94.93 37.78,95.25 70.8,95.25 72.71,93.34 v72.71,76.52
ALUBUS7  (via drill 0.61 pad 1.27)
  Top 0.406: IC17.12 26.67,84.45 27.94,85.72 v27.94,90.17 | v73.98,78.42 79.06,73.34 79.06,64.14 81.92,61.28 IC11.2 81.92,66.67 85.09,69.85 91.76,69.85 93.66,67.94 | 93.66,67.94 94.93,69.22 99.06,69.22 100.01,68.26 100.01,65.09 100.97,64.14 109.86,64.14 115.25,69.53 121.92,69.53 122.87,68.58 122.87,62.23 124.46,60.64 124.46,34.92 123.19,33.66 IC2.11 | IC3.4 93.66,67.94
  Bottom 0.406: v27.94,90.17 30.8,93.03 30.8,95.57 31.43,96.2 71.12,96.2 73.98,93.34 v73.98,78.42 | JP3.8 6.03,78.11 3.49,78.11 2.7,78.9 2.7,85.25 4.45,87 8.26,87 14.61,80.64 20.32,80.64 24.13,84.45 IC17.12
ALUBUS8
  Bottom 0.406: JP3.9 3.81,74.3 1.59,76.52 1.59,85.72 3.81,87.95 9.53,87.95 14.29,83.19 20.64,83.19 23.18,85.72 27.62,85.72 31.43,81.92 IC16.2
ALUBUS9
  Top 0.406: JP3.10 8.57,75.56 11.75,75.56 14.29,78.11 21.27,78.11 23.81,80.64 29.53,80.64 30.8,79.38 IC16.3
ALUBUS10
  Bottom 0.406: JP3.11 6.03,73.03 29.53,73.03 30.8,74.3 IC16.5
ALUBUS11
  Bottom 0.406: JP3.12 IC16.6
ALUBUS12
  Bottom 0.406: JP3.13 6.03,70.48 37.15,70.48 38.42,69.22 IC16.8
ALUBUS13
  Bottom 0.406: JP3.14 9.21,69.22 10.79,67.63 40.96,67.63 42.23,68.9 42.23,70.48 40.96,71.75 IC16.9
ALUBUS14
  Bottom 0.406: JP3.15 6.03,67.94 8.26,67.94 9.53,66.67 42.23,66.67 44.13,68.58 44.13,73.98 41.27,76.83 IC16.11
ALUBUS15
  Top 0.406: IC3.6 98.74,64.77 100.33,63.18 111.12,63.18 112.71,61.59 112.71,44.45 110.17,41.91 110.17,34.92 108.9,33.66 IC8.11
  Bottom 0.406: JP3.16 8.26,65.72 42.55,65.72 45.09,68.26 | IC16.12 41.27,79.38 45.09,75.56 45.09,68.26 | IC3.6 IC3.5 96.2,65.72 95.57,65.09 90.49,65.09 89.85,65.72 89.85,68.26 88.9,69.22 84.77,69.22 81.28,65.72 47.62,65.72 45.09,68.26
ALUOP1  (via drill 0.61 pad 1.27)
  Top 0.406: IC2.1 131.44,20.95 137.79,27.3 137.79,33.97 143.51,39.69 143.51,53.34 144.78,54.61 IC18.9 | IC8.1 112.08,20.95 109.54,23.5 IC8.15 | JP9.6 72.39,6.99 82.87,6.99 v93.66,17.78
  Bottom 0.406: IC2.1 126.36,20.95 123.83,23.5 IC2.15 119.7,23.5 117.16,20.95 IC8.1 | v93.66,17.78 96.84,20.95 103.19,20.95 105.73,23.5 IC8.15
ALURES0
  Top 0.406: IC1.4 111.44,52.07 110.17,53.34 107.63,53.34 106.36,52.07 IC1.2
  Bottom 0.406: JP9.25 47.94,10.48 47.94,19.05 45.09,21.91 45.09,30.48 50.48,35.88 50.48,40.32 54.29,44.13 71.12,44.13 73.66,46.67 103.82,46.67 106.36,49.21 IC1.2
ALURES8  (via drill 0.61 pad 1.27)
  Top 0.406: IC1.3 109.22,50.8 109.22,35.88 108.27,34.92 105.73,34.92 100.65,29.84 89.85,29.84 87.95,27.94 87.95,23.18 84.77,20 82.23,20 79.38,17.14 75.25,17.14 70.48,12.38 v43.18,12.38
  Bottom 0.406: v43.18,12.38 JP9.27
BUSCLKB  (via drill 0.61 pad 1.27)
  Top 0.406: JP10.24 99.06,4.76 100.65,3.17 151.45,3.17 152.72,4.45 152.72,18.1 v151.13,19.68
  Bottom 0.406: v151.13,19.68 126.36,19.68 123.83,22.23 120.02,22.23 117.47,19.68 113.03,19.68 111.12,21.59 111.12,23.18 109.54,24.77 105.09,24.77 102.55,22.23 89.85,22.23 89.22,22.86 89.22,24.13 89.85,24.77 93.03,24.77 93.66,25.4 93.66,27.94 93.03,28.57 IC6.12 89.85,28.57 88.9,29.53 88.9,31.43 89.85,32.38 92.71,32.38 93.66,33.34 93.66,35.24 92.71,36.2 IC6.9
CLK0D
  Bottom 0.406: JP10.17 105.41,9.53 87.63,9.53 81.28,3.17 26.35,3.17 25.08,4.45 6.99,4.45 6.03,5.4 6.03,9.21 1.27,13.97 1.27,36.51 4.45,39.69 8.57,39.69 11.43,42.55 11.43,50.16 15.88,54.61 31.11,54.61 33.02,52.7 IC10.7
F6  (via drill 0.61 pad 1.27)
  Top 0.406: v69.22,46.67 71.75,49.21 IC11.9
  Bottom 0.406: IC5.8 37.15,20.95 40.01,23.81 40.01,36.2 41.27,37.47 47.31,37.47 48.58,38.73 48.58,41.27 53.34,46.04 68.58,46.04 v69.22,46.67
F7  (via drill 0.61 pad 1.27)
  Top 0.406: v70.8,46.04 73.03,48.26 73.03,55.56 74.3,56.83 IC11.5
  Bottom 0.406: IC5.9 37.15,18.41 40.96,22.23 40.96,34.29 41.59,34.92 48.26,34.92 49.53,36.2 49.53,40.64 53.98,45.09 69.85,45.09 v70.8,46.04
FC  (via drill 0.61 pad 1.27)
  Top 0.406: IC5.2 36.83,36.2 40.64,32.38 v50.16,32.38
  Bottom 0.406: IC5.2 33.34,36.2 31.75,37.78 31.75,52.39 30.48,53.66 24.45,53.66 22.86,52.07 IC10.3 | v50.16,32.38 50.16,24.77 51.75,23.18 51.75,15.24 53.66,13.34 122.56,13.34 125.73,10.16 125.73,6.99 JP10.2
FN  (via drill 0.61 pad 1.27)
  Top 0.406: IC5.4 36.83,31.11 40.64,27.3 v47.62,27.3
  Bottom 0.406: IC5.4 33.34,31.11 29.53,34.92 29.53,45.09 27.94,46.67 IC10.5 | v47.62,27.3 47.62,24.77 49.85,22.54 49.85,14.61 53.02,11.43 118.43,11.43 120.65,9.21 120.65,6.99 JP10.6
FV  (via drill 0.61 pad 1.27)
  Top 0.406: v26.04,48.26 29.53,48.26 30.48,49.21 IC10.6 | IC5.5 36.83,28.57 40.64,24.77 v46.35,24.77
  Bottom 0.406: IC5.5 33.34,28.57 28.57,33.34 28.57,44.13 26.04,46.67 v26.04,48.26 | v46.35,24.77 48.9,22.23 48.9,14.29 52.7,10.48 116.84,10.48 118.11,9.21 118.11,6.99 JP10.8
FZ  (via drill 0.61 pad 1.27)
  Top 0.406: IC5.3 36.83,33.66 40.64,29.84 v48.9,29.84
  Bottom 0.406: IC5.3 33.34,33.66 30.48,36.51 30.48,46.04 29.21,47.31 29.21,52.07 28.57,52.7 26.04,52.7 25.4,52.07 IC10.4 | v48.9,29.84 48.9,24.77 50.8,22.86 50.8,14.92 53.34,12.38 120.33,12.38 123.19,9.53 123.19,6.99 JP10.4
GND
  Top 0.406: IC3.3 91.12,67.94 90.17,68.9 87,68.9 86.04,67.94 IC3.1
  Bottom 0.406: C1.2 22.54,14.92 22.54,19.68 23.81,20.95 IC14.2 | IC13.10 58.1,15.88 59.37,17.14 67.63,17.14 69.22,15.56 C10.2
  pour Bottom (isolate 0.61): 0,100.01 160.02,100.01 160.02,0 0,0
  pour Top (isolate 0.61): 0,100.01 160.02,100.01 160.02,0 0,0
LBUS7  (via drill 0.61 pad 1.27)
  Top 0.406: v120.97,47.62 122.24,46.35 IC2.9
  Bottom 0.406: v120.97,47.62 109.54,47.62 107.63,49.53 107.63,52.39 106.68,53.34 96.84,53.34 96.2,53.98 45.4,53.98 43.81,55.56 14.61,55.56 7.94,48.9 JP5.10
LBUS15  (via drill 0.61 pad 1.27)
  Top 0.406: v99.69,54.61 99.69,50.16 107,42.86 IC8.9
  Bottom 0.406: v99.69,54.61 99.38,54.93 46.04,54.93 44.45,56.52 15.24,56.52 12.7,59.05 JP5.2
LOAD_FLAGS0  (via drill 0.61 pad 1.27)
  Top 0.406: IC3.14 91.12,73.34 91.76,72.71 120.97,72.71 121.6,73.34 IC4.14 | IC7.1 85.09,18.73 88.9,22.54 88.9,26.35 89.85,27.3 108.9,27.3 111.44,29.84 111.44,41.27 115.25,45.09 115.25,54.29 116.52,55.56 IC1.11 | v83.5,14.92 78.42,9.84 50.48,9.84 49.53,8.89 49.53,6.99 JP9.24
  Bottom 0.406: IC1.11 122.87,65.09 122.87,72.07 121.6,73.34 IC4.14 | IC7.1 v83.5,14.92
LOAD_FLAGS1  (via drill 0.61 pad 1.27)
  Top 0.406: IC1.10 IC4.2 | IC7.2 84.45,21.27 86.68,23.5 86.68,28.26 87.63,29.21 87.63,62.55 88.58,63.5 IC3.2 | JP9.26 45.72,5.08 46.67,4.13 81.6,4.13 87.95,10.48 89.22,10.48 v93.34,14.61
  Bottom 0.406: IC3.2 88.58,65.72 90.17,64.14 117.47,64.14 119.06,65.72 IC4.2 | IC7.2 90.17,14.61 v93.34,14.61
N$1
  Top 0.406: IC8.5 118.11,31.11 119.38,32.38 123.83,32.38 125.41,33.97 125.41,49.21 126.68,50.48 IC4.5
  Bottom 0.406: IC4.5 IC4.6
N$2
  Bottom 0.406: IC18.4 139.7,51.44 135.89,55.24 113.03,55.24 111.44,56.83 IC1.13
N$3
  Bottom 0.406: IC18.2 134.62,51.44 131.76,54.29 111.12,54.29 108.9,56.52 IC1.14 IC1.15
N$6
  Bottom 0.406: IC16.1 34.92,87 46.35,87 50.48,82.87 IC15.1
N$7
  Bottom 0.406: IC15.2 58.1,80.96 56.52,79.38 51.12,79.38 47.31,83.19 38.42,83.19 36.2,80.96 36.2,78.11 34.92,76.83 IC16.4 33.66,76.83
N$8
  Bottom 0.406: IC15.4 63.18,84.77 63.82,85.41 66.36,85.41 66.99,84.77 66.99,80.96 63.5,77.47 45.09,77.47 41.91,80.64 38.73,80.64 37.15,79.06 37.15,75.88 38.73,74.3 IC16.10
N$9
  Bottom 0.406: IC15.5 65.72,82.55 61.59,78.42 50.48,78.42 46.99,81.92 IC16.13
N$10  (via drill 0.61 pad 1.27)
  Top 0.406: IC17.1 20,91.76 30.48,91.76 v32.38,93.66
  Bottom 0.406: v32.38,93.66 66.67,93.66 68.26,92.08 IC15.9
N$11  (via drill 0.61 pad 1.27)
  Top 0.406: v31.75,87.95 26.99,83.19 20,83.19 18.73,81.92 IC17.4
  Bottom 0.406: IC15.10 65.72,91.12 64.14,92.71 60.01,92.71 59.37,92.08 59.37,89.22 53.98,83.82 50.8,83.82 46.67,87.95 v31.75,87.95
N$12
  Bottom 0.406: IC15.12 60.64,89.22 56.83,85.41 56.83,81.28 55.88,80.33 51.44,80.33 46.04,86.04 36.51,86.04 34.92,84.45 34.92,81.6 33.97,80.64 29.53,80.64 28.26,79.38 IC17.10
N$13
  Bottom 0.406: IC17.13 28.26,87 33.97,92.71 56.52,92.71 58.1,91.12 IC15.13
N$14  (via drill 0.61 pad 1.27)
  Top 0.406: IC15.6 68.26,84.14 69.85,85.72 v79.69,85.72
  Bottom 0.406: v79.69,85.72 82.55,82.87 IC20.1 88.58,81.28 92.39,77.47 92.39,73.34 93.34,72.39 97.79,72.39 98.74,73.34 IC3.11
N$15  (via drill 0.61 pad 1.27)
  Top 0.406: IC15.8 v79.69,90.49
  Bottom 0.406: v79.69,90.49 82.87,87.31 88.9,87.31 91.12,85.09 IC20.2 91.12,80.96 96.2,75.88 IC3.12
N$16
  Bottom 0.406: IC3.10 101.28,75.88 99.06,78.11 95.25,78.11 93.66,79.69 IC20.3
N$17
  Top 0.406: IC10.9 40.64,63.5 58.1,63.5 64.14,57.47 64.14,55.56 66.99,52.7 66.99,45.09 73.34,38.73 73.34,28.26 75.25,26.35 IC7.11
  Bottom 0.406: IC10.10 IC10.9
N$19
  Top 0.406: IC4.4 124.14,67.94 125.41,69.22 127,69.22 127.95,68.26 127.95,50.48 126.36,48.9 126.36,32.7 127.95,31.11 IC2.5
N$21
  Top 0.406: IC18.8 147.32,59.05 146.37,60.01 141.92,60.01 140.97,59.05 140.97,47.31 134.94,41.27 134.94,29.53 131.44,26.04 IC2.3
  Bottom 0.406: IC2.3 126.36,26.04 123.83,28.57 IC2.13 121.92,28.89 120.02,28.89 117.16,26.04 IC8.3 112.08,26.04 109.54,28.57 IC8.13
N$32  (via drill 0.61 pad 1.27)
  Top 0.406: v61.59,63.5 60.64,64.45 IC9.4
  Bottom 0.406: IC10.14 22.86,59.69 26.67,63.5 v61.59,63.5
N$48  (via drill 0.61 pad 1.27)
  Top 0.406: v65.41,62.23 68.26,65.09 IC9.7
  Bottom 0.406: v65.41,62.23 27.94,62.23 25.4,59.69 IC10.13
N$49  (via drill 0.61 pad 1.27)
  Top 0.406: v67.31,62.23 69.53,64.45 69.53,72.07 70.8,73.34 IC9.9
  Bottom 0.406: v67.31,62.23 66.04,60.96 29.21,60.96 27.94,59.69 IC10.12
N$50
  Top 0.406: IC10.11 30.48,59.05 38.1,66.67 48.26,66.67 52.7,71.12 65.09,71.12 66.99,73.03 66.99,76.83 66.04,77.79 64.14,77.79 63.18,76.83 IC9.12
N$51
  Bottom 0.406: IC7.3 IC7.12
N$52  (via drill 0.61 pad 1.27)
  Top 0.406: v65.41,57.15 67.94,54.29 67.94,45.72 74.93,38.73 v77.15,38.73
  Bottom 0.406: IC12.3 53.34,57.47 53.98,56.83 65.09,56.83 v65.41,57.15 | v77.15,38.73 IC6.8
N$53  (via drill 0.61 pad 1.27)
  Top 0.406: v96.84,49.21 96.84,33.02 94.93,31.11 IC6.11
  Bottom 0.406: IC12.11 50.8,52.07 51.75,53.02 69.85,53.02 70.48,52.39 70.48,49.85 71.12,49.21 v96.84,49.21
N$54
  Bottom 0.406: IC7.6 86.68,31.43 88.9,33.66 IC6.10
N$55
  Bottom 0.406: IC7.8 77.79,33.97 81.6,30.16 85.72,30.16 89.85,26.04 IC6.13
OP0
  Bottom 0.406: JP7.9 151.45,39.69 148.27,42.86 74.93,42.86 72.39,40.32 55.56,40.32 54.29,39.05 54.29,34.29 54.93,33.66 IC13.3
OP1
  Bottom 0.406: JP7.8 151.76,42.23 150.18,43.81 74.61,43.81 72.07,41.27 55.24,41.27 53.34,39.37 53.34,32.7 54.93,31.11 IC13.4
OP2
  Bottom 0.406: JP7.7 74.3,44.77 71.75,42.23 54.93,42.23 52.39,39.69 52.39,31.11 54.93,28.57 IC13.5
OP3
  Bottom 0.406: JP7.6 152.08,47.31 150.5,45.72 73.98,45.72 71.44,43.18 54.61,43.18 51.44,40.01 51.44,29.53 54.93,26.04 IC13.6
RBUS0
  Top 0.406: IC13.18 60.33,33.66 59.05,34.92 52.39,34.92 51.12,33.66 IC5.18 40.64,33.66 36.83,37.47 30.8,37.47 28.26,40.01 11.11,40.01 JP4.1
RBUS1
  Top 0.406: IC13.17 60.33,31.11 59.05,32.38 52.39,32.38 51.12,31.11 IC5.17 40.64,31.11 36.83,34.92 30.8,34.92 28.26,37.47 11.11,37.47 JP4.2
RBUS2
  Top 0.406: IC13.16 60.33,28.57 59.05,29.84 52.39,29.84 51.12,28.57 IC5.16 40.64,28.57 36.83,32.38 30.8,32.38 28.26,34.92 13.34,34.92 10.79,32.38 6.03,32.38 JP4.3
RBUS3
  Top 0.406: IC13.15 60.33,26.04 59.05,27.3 52.39,27.3 51.12,26.04 IC5.15 40.64,26.04 36.83,29.84 30.8,29.84 28.26,32.38 12.38,32.38 11.11,31.11 JP4.4
RBUS4
  Top 0.406: IC13.14 60.33,23.5 59.05,24.77 52.07,24.77 50.8,23.5 IC5.14 40.64,23.5 36.83,27.3 30.8,27.3 28.26,29.84 6.03,29.84 JP4.5
RBUS5
  Top 0.406: IC13.13 60.33,20.95 59.05,22.23 47.62,22.23 46.35,20.95 IC5.13 40.64,20.95 36.83,24.77 30.8,24.77 28.26,27.3 12.38,27.3 11.11,28.57 JP4.6
RBUS6
  Top 0.406: IC13.12 60.33,18.41 59.05,19.68 46.35,19.68 45.09,18.41 IC5.12 40.64,18.41 36.83,22.23 30.8,22.23 28.26,24.77 13.34,24.77 10.79,27.3 6.03,27.3 JP4.7
RBUS7  (via drill 0.61 pad 1.27)
  Top 0.406: JP4.8 10.16,26.04 13.97,22.23 27.94,22.23 30.48,19.68 36.83,19.68 40.64,15.88 IC5.11 47.94,15.88 49.21,17.14 59.05,17.14 60.33,15.88 IC13.11 65.09,15.88 66.67,17.46 66.67,25.72 68.9,27.94 v68.9,35.88 | v79.69,40.01 v79.69,35.88
  Bottom 0.406: IC2.10 119.7,36.2 118.43,37.47 96.2,37.47 93.66,40.01 v79.69,40.01 | v79.69,35.88 v68.9,35.88
RBUS8
  Bottom 0.406: JP4.9 6.03,22.23 13.02,22.23 14.29,23.5 IC14.18
RBUS9
  Bottom 0.406: JP4.10 12.38,23.5 14.92,26.04 IC14.17
RBUS10
  Bottom 0.406: JP4.11 6.03,19.68 18.1,19.68 19.68,21.27 19.68,27.3 18.41,28.57 IC14.16
RBUS11
  Bottom 0.406: JP4.12 13.65,20.95 14.92,22.23 18.1,22.23 18.73,22.86 18.73,26.67 18.1,27.3 15.24,27.3 14.29,28.26 14.29,30.16 15.24,31.11 IC14.15
RBUS12
  Bottom 0.406: JP4.13 6.03,17.14 8.26,17.14 9.53,15.88 18.1,15.88 21.59,19.37 21.59,31.43 19.37,33.66 IC14.14
RBUS13
  Bottom 0.406: IC14.13 15.24,36.2 14.29,35.24 14.29,33.34 15.24,32.38 19.37,32.38 20.64,31.11 20.64,19.68 17.78,16.83 9.84,16.83 8.26,18.41 JP4.14
RBUS14
  Bottom 0.406: JP4.15 3.17,17.46 3.17,34.92 4.45,36.2 13.65,36.2 16.19,38.73 IC14.12
RBUS15  (via drill 0.61 pad 1.27)
  Top 0.406: v67.94,37.47 62.23,37.47 55.24,44.45 26.99,44.45 25.4,42.86 18.41,42.86 IC14.11
  Bottom 0.406: v67.94,37.47 93.66,37.47 96.2,34.92 102.55,34.92 103.82,36.2 IC8.10 | JP4.16 6.03,14.61 3.49,14.61 2.22,15.88 2.22,35.56 3.81,37.15 12.06,37.15 16.19,41.27 IC14.11
RST  (via drill 0.61 pad 1.27)
  Top 0.406: v151.45,13.65 151.45,5.4 150.18,4.13 118.75,4.13 118.11,4.76 118.11,6.99 JP10.9
  Bottom 0.406: IC10.15 20.32,59.69 25.4,64.77 74.61,64.77 76.2,63.18 113.98,63.18 115.25,61.91 115.25,57.15 116.2,56.2 123.19,56.2 130.49,63.5 154.31,63.5 157.8,60.01 157.8,20 v151.45,13.65

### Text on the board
Top: #3
tsilk: VCC2 | GND1 | IC17 | 74LS02N | JP3 | IC16 | 74LS21N | 74LS08N | 74LS02N | IC15 | IC20 | 74LS157N | 74LS153N | 74LS153N | IC9 | IC3 | IC4 | JP7 | JP5 | IC12 | IC11 | 74LS74N | 74LS74N | 74LS173N | 74LS151N | 74LS04N | IC10 | IC1 | IC18 | IC5 | IC13 | 74LS541N | 74LS541N | JP4 | JP2 | 74LS32N | IC6 | 74LS151N | 74LS151N | 74LS541N | 74LS08N | IC8 | IC2 | IC14 | IC7 | GND2 | VCC1 | 10u | JP9 | JP10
